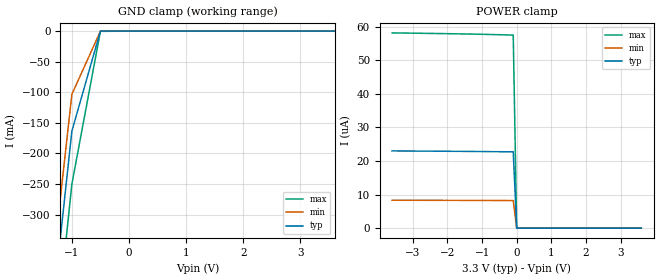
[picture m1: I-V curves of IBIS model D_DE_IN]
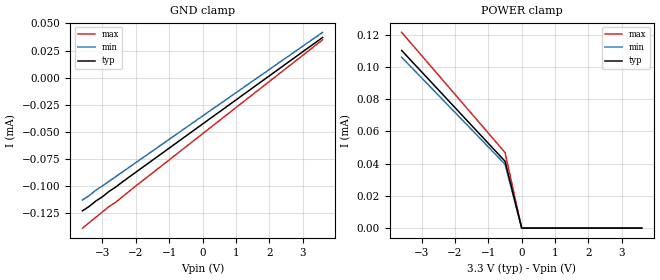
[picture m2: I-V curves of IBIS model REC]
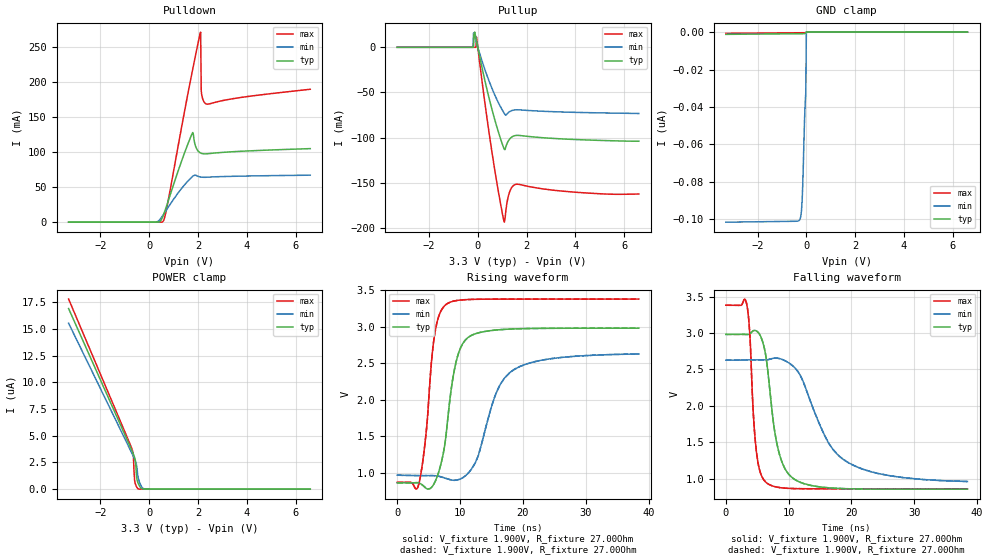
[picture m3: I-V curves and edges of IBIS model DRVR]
| Texas Instruments Incorporated
| 3.3v Full-Duplex RS-485 Drivers and Receivers
| Model valid for speed grades upto 26Mbps(13MHz Clock frequency)
| Marketing part#   Voltage Range   Package-type   Temperature
| SN65HVD30DR   3.0V - 3.6V   SOIC (D) 8-pin  -40C to 85C
[IBIS Ver]   4.0
[Comment char]   |_char
[File name]   sn65hvd30.ibs
[File Rev]   1.1
[Date]   03/16/2009
[Source]   File originated at Texas Instruments Incorporated.
   Data Transmission Products Group.
[Notes]   Revision History:
   Rev 1.0: 03/29/2007
   - Initial version built by Data Transmission group
   Rev 1.1: 02/18/2009
   - Updated Disclaimer
   - updated IBIS ver to 4.0
   - Updated DRVR and RECEIVER_OUT model characteristics
   - Updated ccomp for RECEIVER_OUT
   - RECEIVER_OUT ccomp is based on PVT conditions, ignore warnings
   - RECEIVER_OUT and DRVR pullup and pulldown non-montonicity reflects
   true buffer behavior
[Disclaimer] This product is designed as an aid for customers of Texas Instruments.
   No warranties, either expressed or implied, with respect to this third
   party software (if any) or with respect to its fitness for any
   particular purpose is claimed by Texas Instruments or the author. The
   software (if any) is provided solely on an "as is" basis. The entire
   risk as to its quality and performance is with the customer
[Copyright]   Copyright 2009 Texas Instruments Incorporated. All rights reserved.
[Component]   SN65HVD30DR
[Manufacturer]  Texas Instruments Incorporated
[Package]   |SOIC (D) 8-pin
|   typ   min   max
R_pkg   0.071   0.050   0.091
L_pkg   2.203nH   1.540nH   2.930nH
C_pkg   0.465pF   0.385pF   0.609pF
[Pin]   signal_name   model_name   R_pin   L_pin   C_pin
1   VCC   POWER   0.091   2.615n   0.500p
2   R   RECEIVER_OUT   0.076   2.346n   0.483p
3   D   D_DE_IN   0.062   1.755n   0.395p
4   GND   GND   0.090   2.593n   0.498p
5   Y   DRVR   0.073   2.300n   0.480p
6   Z   DRVR   0.076   2.012n   0.407p
7   B   REC   0.050   1.540n   0.385p
8   A   REC   0.070   1.897n   0.412p
[Diff_pin]   inv_pin   vdiff   tdelay_typ   tdelay_min   tdelay_max
| The 'A' pin is Diff_pin and the 'B' pin is the inv_pin
5   6   0.200   0 0 0
7   8   0.200   0 0 0
| Models and submodels in the file (4): D_DE_IN (Input), REC (Input), DRVR (I/O), RECEIVER_OUT (Output)
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|   Driver Input / Driver Enable / Model
[Model]   D_DE_IN
Model_type   Input
|Signals   D
Vinh = 2.0
Vinl = 0.8
|   typ   min   max
C_comp   23pF   19pF   27pF
|   typ   min   max
[Temperature Range]   27   -40   85
[Voltage range]   3.3V   3.0V   3.6V
[GND_clamp]
|   Voltage   I(typ)   I(min)   I(max)
-3.6V     -2.348A    -2.232A    -2.506A
-1.5V     -596.3mA   -523.6mA   -696.4mA
-1V       -163.5mA   -103.3mA   -250mA
-500mV    -12.8uA    -27.56uA   -399.4uA
3.6V      22.76uA    57.48uA    8.245uA
[Power_clamp]
| Note that the[POWER_clamp]voltage table is referenced to Vcc
| and is calculated using Vtable=Vcc - Vmeasured.
|   Voltage   I(typ)   I(min)   I(max)
-3.6V     23.01uA    8.325uA    58.18uA
-100mV    22.74uA    8.227uA    57.52uA
0V        0A         0A         0A
3.6V      0A         0A         0A
|   Receiver Input / Model
[Model]   REC
Model_type   Input
|Signals   A,B
Vinh = 2.0
Vinl = 0.8
|   typ   min   max
C_comp   3pF   2.5pF   3.5pF
|   typ   min   max
[Temperature Range]   27   -40   85
[Voltage range]   3.3V   3.0V   3.6V
[GND_clamp]
|   Voltage   I(typ)   I(min)   I(max)
-3.6V     -123uA     -113uA     -139uA
-2.8V     -105uA     -95.7uA    -119uA
-2.6V     -101uA     -91.4uA    -115uA
3.6V      37.1uA     41.8uA     34.9uA
[Power_clamp]
| Note that the[POWER_clamp]voltage table is referenced to Vcc
| and is calculated using Vtable=Vcc - Vmeasured.
|   Voltage   I(typ)   I(min)   I(max)
-3.6V     110.3uA    106.1uA    121.5uA
-3.3V     103.6uA    99.69uA    114.3uA
-3V       96.98uA    93.26uA    107.1uA
-2.5V     85.89uA    82.54uA    95.07uA
-2V       74.79uA    71.82uA    83.04uA
-1.5V     63.7uA     61.1uA     71uA
-1V       52.6uA     50.38uA    58.96uA
-500mV    41.51uA    39.65uA    46.93uA
0V        0A         0A         0A
3.6V      0A         0A         0A
|   Driver Output / Receiver Input Model
[Model]   DRVR
Model_type   I/O
| Signals   Y,Z
Vinl = 0.9V
Vinh = 2.8V
Vmeas = 1.7V   |Reference voltage for timing measurements
Cref = 50pF   |Timing specification test load capacitance value
Rref = 54Ohm   |Note: 54 Ohm load; single-ended configuration
|   Timing specification test load voltage
| variable   typ   min   max
C_comp   28pF   24pF   32pF
|   typ   min   max
[Temperature Range]   40.0   -40   40
[Voltage range]   3.3V   3.0V   3.6V
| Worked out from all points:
|   slope of the pulldown table from 0 to 0.495 V, typ, clamps not added: 150 ohm
|   slope of the pullup table from 0 to 0.495 V, typ, clamps not added: 8.27 ohm
|   falling waveform, V_fixture 1.900V, R_fixture 27.00Ohm: 20-80 % time 2.15ns typ, 5.78ns min, 988ps max; typ from 2.98 V to 0.858 V
|   rising waveform, V_fixture 1.900V, R_fixture 27.00Ohm: 20-80 % time 2.1ns typ, 3.94ns min, 1.55ns max; typ from 0.858 V to 2.98 V
|   rising waveform, V_fixture 1.900V, R_fixture 27.00Ohm: 20-80 % time 2.1ns typ, 3.94ns min, 1.55ns max; typ from 0.858 V to 2.98 V
|   falling waveform, V_fixture 1.900V, R_fixture 27.00Ohm: 20-80 % time 2.15ns typ, 5.78ns min, 988ps max; typ from 2.98 V to 0.858 V
[Pulldown]
|   Voltage   I(typ)   I(min)   I(max)
-3.3V     -1.965pA   -685.2pA   -1.411pA
272.9mV   4.077uA    165uA      1.782nA
570.7mV   9.035mA    10.12mA    1.19mA
744.4mV   26.41mA    19.33mA    24.32mA
1.762V    126.6mA    64.88mA    214.5mA
1.811V    125.4mA    66.17mA    223.2mA
1.935V    105.6mA    66.55mA    244.3mA
2.109V    98.77mA    64.53mA    271.5mA
2.134V    98.39mA    64.4mA     186.9mA
2.208V    97.72mA    64.17mA    174.6mA
2.332V    97.6mA     64.17mA    169mA
6.6V      105.1mA    67.15mA    189.8mA
[GND Clamp]
|   Voltage   I(typ)   I(min)   I(max)
-3.3V     -1.206nA   -101.5nA   -666.8pA
-397mV    -899pA     -101nA     -372pA
-248.1mV  -883.1pA   -99.46nA   -356.9pA
-223.3mV  -880.3pA   -97.98nA   -354.4pA
-198.5mV  -877.1pA   -95.15nA   -351.9pA
-173.7mV  -873.1pA   -90.1nA    -349.4pA
-148.9mV  -867.3pA   -81.98nA   -346.8pA
-74.44mV  -801.4pA   -47.05nA   -339.3pA
-49.62mV  -732.3pA   -38.53nA   -336.8pA
-24.81mV  -622.9pA   -32.89nA   -334.3pA
0V        0A         0A         0A
6.6V      0A         0A         0A
[Pullup]
|   Voltage   I(typ)   I(min)   I(max)
-3.3V     2.229uA    1.936uA    2.571uA
-198.5mV  2.099uA    1.938uA    2.347uA
-173.7mV  2.09uA     15.93mA    2.344uA
-148.9mV  14.5mA     13.65mA    2.34uA
-124.1mV  16.86mA    11.37mA    2.335uA
-74.44mV  10.15mA    6.844mA    2.223uA
-49.62mV  6.813mA    4.598mA    11.34mA
545.9mV   -65.06mA   -43.09mA   -109.7mA
1.092V    -113mA     -73.41mA   -193.7mA
1.29V     -102.2mA   -71.55mA   -161.4mA
1.563V    -97.66mA   -69.24mA   -151.8mA
6.6V      -104mA     -73.31mA   -162.5mA
[POWER Clamp]
|   Voltage   I(typ)   I(min)   I(max)
-3.3V     16.91uA    15.54uA    17.8uA
-694.7mV  3.541uA    3.298uA    3.694uA
-645.1mV  3.269uA    3.056uA    3.129uA
-620.3mV  3.123uA    2.931uA    1.666uA
-595.5mV  2.961uA    2.801uA    809.5nA
-570.7mV  2.754uA    2.663uA    525.1nA
-545.9mV  2.213uA    2.509uA    383.7nA
-521.1mV  1.282uA    2.315uA    254.1nA
-471.4mV  668.3nA    1.343uA    70.95nA
-322.6mV  79.17nA    276nA      900.6pA
-148.9mV  1.263nA    18.84nA    288.1pA
6.6V      0A         0A         0A
[Ramp]
R_load = 27.00Ohm
|   typ   min   max
dV/dt_r   1.273V/2.121ns   998.279mV/3.944ns   1.510V/1.549ns
dV/dt_f   1.273V/2.152ns   998.279mV/5.803ns   1.510V/992.120ps
[Falling Waveform]
V_fixture = 1.900V
V_fixture_min = 1.795V
V_fixture_max = 2.120V
R_fixture = 27.00Ohm
|   Time   V(typ)   V(min)   V(max)
0s        2.981V     2.627V     3.381V
3.303ns   2.98V      2.63V      3.406V
3.782ns   2.985V     2.631V     3.035V
4.364ns   3.03V      2.631V     1.918V
4.851ns   3.029V     2.631V     1.386V
6.553ns   2.576V     2.632V     940.8mV
8.309ns   1.415V     2.653V     883.8mV
10.93ns   993.4mV    2.527V     866.4mV
18.67ns   866.2mV    1.268V     863.8mV
38.46ns   858.4mV    963.2mV    863.8mV
[Rising Waveform]
V_fixture = 1.900V
V_fixture_min = 1.795V
V_fixture_max = 2.120V
R_fixture = 27.00Ohm
|   Time   V(typ)   V(min)   V(max)
0s        858.4mV    963.2mV    863.7mV
3.427ns   856.8mV    957.9mV    838.2mV
4.538ns   786.7mV    957.2mV    1.49V
5.944ns   859.5mV    956mV      2.886V
7.807ns   1.539V     917.9mV    3.308V
9.479ns   2.555V     896.7mV    3.361V
11.84ns   2.884V     1.051V     3.376V
15.72ns   2.956V     2.086V     3.38V
18.67ns   2.971V     2.417V     3.38V
38.46ns   2.981V     2.627V     3.38V
[Rising Waveform]
V_fixture = 1.900V
V_fixture_min = 1.795V
V_fixture_max = 2.120V
R_fixture = 27.00Ohm
|   Time   V(typ)   V(min)   V(max)
0s        858.4mV    963.2mV    863.7mV
3.427ns   856.8mV    957.9mV    838.2mV
4.538ns   786.7mV    957.2mV    1.49V
5.944ns   859.5mV    956mV      2.886V
7.807ns   1.539V     917.9mV    3.308V
9.479ns   2.555V     896.7mV    3.361V
11.84ns   2.884V     1.051V     3.376V
15.72ns   2.956V     2.086V     3.38V
18.67ns   2.971V     2.417V     3.38V
38.46ns   2.981V     2.627V     3.38V
[Falling Waveform]
V_fixture = 1.900V
V_fixture_min = 1.795V
V_fixture_max = 2.120V
R_fixture = 27.00Ohm
|   Time   V(typ)   V(min)   V(max)
0s        2.981V     2.627V     3.381V
3.303ns   2.98V      2.63V      3.406V
3.782ns   2.985V     2.631V     3.035V
4.364ns   3.03V      2.631V     1.918V
4.851ns   3.029V     2.631V     1.386V
6.553ns   2.576V     2.632V     940.8mV
8.309ns   1.415V     2.653V     883.8mV
10.93ns   993.4mV    2.527V     866.4mV
18.67ns   866.2mV    1.268V     863.8mV
38.46ns   858.4mV    963.2mV    863.8mV
